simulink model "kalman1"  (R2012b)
settings: Solver=ode45  StartTime=0.0  StopTime=10.0  RelTol=1e-3
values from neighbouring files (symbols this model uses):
  A = [0 1 0 0 0 0    [beobachter_1.m]    (also in beobachter_2.m; beobachter_22.m; kalman_1.m = my_sys.a; kalman_10.m = my_sys.a)
  B = [0 1 0 0 0 0]'    [beobachter_1.m]    (also in beobachter_2.m; beobachter_22.m; kalman_1.m = my_sys.b; kalman_10.m = my_sys.b)
  C = [0 0 0 0 1 0]    [beobachter_1.m]    (also in beobachter_2.m; beobachter_22.m; kalman_1.m = my_sys.c; kalman_10.m = my_sys.c)
  dtn = 0.01    [kalman_1.m]    (also in kalman_10.m; kalman_11.m; kalman_12.m; kalman_d1.m)
  G = eye(2,2)    [kalman_1.m]    (also in kalman_10.m; kalman_11.m; kalman_12.m; kalman_d1.m = eye(3,3))
  vnd = 1e-4    (= 0.0001)    [kalman_1.m]    (also in kalman_10.m; kalman_11.m; kalman_12.m; kalman_13.m = 0.01)
  vny = 1e-6    (= 1e-06)    [kalman_1.m]    (also in kalman_10.m; kalman_11.m = ', num2str(vny),' )']); kalman_12.m = ', num2str(vny),' )']); kalman_13.m = ', num2str(vny),' )']))
undefined symbols (not defined in the file or in its folder): L
libraries: simulink x2

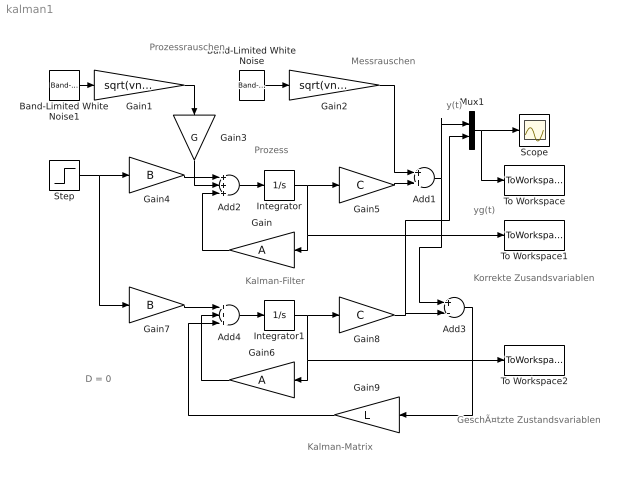
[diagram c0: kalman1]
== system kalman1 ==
  note: D = 0
  note: Kalman-Matrix
  note: Kalman-Filter
  note: Prozess
  note: Messrauschen
  note: Prozessrauschen
  note: yg(t)
  note: y(t)
  note: GeschÃ¤tzte Zustandsvariablen
  note: Korrekte Zusandsvariablen
  Add1 : Sum
  Add2 : Sum  Inputs=+++
  Add3 : Sum  Inputs=+-
  Add4 : Sum  Inputs=+++
  Band-Limited White Noise : simulink/Sources/Band-Limited White Noise  Cov=[dtn]  Ts=dtn  seed=[23341]
  Band-Limited White Noise1 : simulink/Sources/Band-Limited White Noise  Cov=[dtn, dtn]  Ts=[dtn]  seed=[296441, 32786]
  Gain : Gain  Gain=A  Multiplication=Matrix(K*u)
  Gain1 : Gain  Gain=sqrt(vnd/dtn)
  Gain2 : Gain  Gain=sqrt(vny/dtn)
  Gain3 : Gain  Gain=G  Multiplication=Matrix(K*u)
  Gain4 : Gain  Gain=B  Multiplication=Matrix(K*u)
  Gain5 : Gain  Gain=C  Multiplication=Matrix(K*u)
  Gain6 : Gain  Gain=A  Multiplication=Matrix(K*u)
  Gain7 : Gain  Gain=B  Multiplication=Matrix(K*u)
  Gain8 : Gain  Gain=C  Multiplication=Matrix(K*u)
  Gain9 : Gain  Gain=L  Multiplication=Matrix(K*u)
  Integrator : Integrator
  Integrator1 : Integrator
  Mux1 : Mux  Inputs=2
  Scope : Scope
  Step : Step  SampleTime=0
  To Workspace : ToWorkspace  VariableName=y  SaveFormat=Structure With Time
  To Workspace1 : ToWorkspace  VariableName=y1  SaveFormat=Structure With Time
  To Workspace2 : ToWorkspace  VariableName=y2  SaveFormat=Structure With Time
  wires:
  Band-Limited White Noise/1 -> Gain2/1
  Gain2/1 -> Add1/1
  Add1/1 -> Add3/1, Mux1/1
  Add2/1 -> Integrator/1
  Step/1 -> Gain7/1, Gain4/1
  Band-Limited White Noise1/1 -> Gain1/1
  Gain1/1 -> Gain3/1
  Gain/1 -> Add2/3
  Gain3/1 -> Add2/2
  Gain4/1 -> Add2/1
  Gain5/1 -> Add1/2
  Integrator1/1 -> Gain8/1, Gain6/1, To Workspace2/1
  Add4/1 -> Integrator1/1
  Gain7/1 -> Add4/1
  Gain6/1 -> Add4/2
  Gain9/1 -> Add4/3
  Add3/1 -> Gain9/1
  Integrator/1 -> To Workspace1/1, Gain/1, Gain5/1
  Gain8/1 -> Mux1/2, Add3/2
  Mux1/1 -> Scope/1, To Workspace/1
